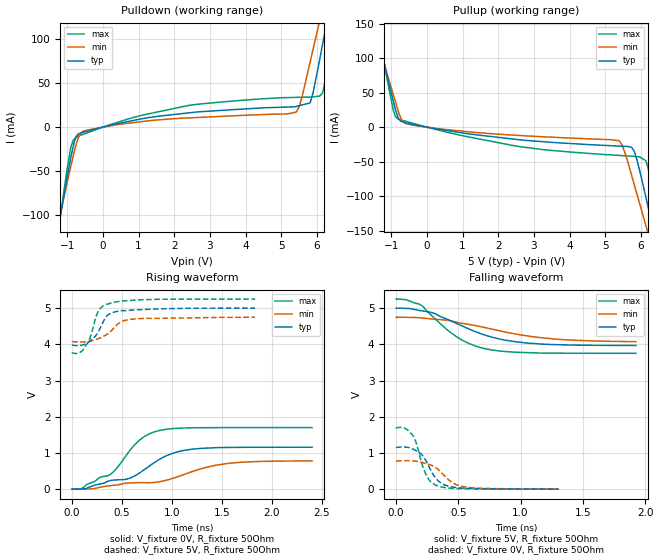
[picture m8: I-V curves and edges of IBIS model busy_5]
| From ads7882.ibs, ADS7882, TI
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|   busy_5 Model
[Model]   busy_5
Model_type   Output
Polarity   Non-Inverting
Vmeas = 2.5
Vref = 2.5
Cref = 20pF
Rref = 50
|   typ   min   max
|   (nom PVT)   (Fast PVT)   (slow PVT)
|C_comp from frequency sweep method (F=1.5MHz)
C_comp   1.072e-12   9.914e-13   1.154e-12
|ON state : BUFFER OUTPUT TURNED HIGH
|C_comp   1.072e-12   9.914e-13   1.154e-12
|OFF state: BUFFER OUTPUT TURNED LOW
|C_comp   1.063e-12   9.642e-13   1.166e-12
|C_comp from LC tank measurement(L=1nH)
|Resonant Frequency(Hz)   6.060e+09   6.040e+09   6.110e+09
|C_comp   6.904e-13   6.950e-13   6.792e-13
|ON state : BUFFER OUTPUT TURNED HIGH
|Resonant Frequency(Hz)   6.060e+09   6.040e+09   6.110e+09
|C_comp   6.904e-13   6.950e-13   6.792e-13
|OFF state: BUFFER IN HIGH IMPEDANCE
|Resonant Frequency   6.010e+09   6.060e+09   5.410e+09
|C_comp   7.020e-13   6.905e-13   8.663e-13
| Where nom  PVT is Nominal Process,  5V,  25C
|   Fast PVT is Strong Process,   5.25V,  -40C
|   Slow PVT is Weak Process,   4.75V,  85C
[Voltage Range]   5   4.75   5.25
|Ambient Temperature   25   85   -40
|Junction Temperature
[Temperature Range]   25   85   -40
[Pullup Reference]   5   4.75   5.25
[Pulldown Reference]   0   0   0
[Power Clamp Reference]   5   4.75   5.25
[GND Clamp Reference]   0   0   0
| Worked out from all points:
|   slope of the pulldown table from 0 to 0.75 V, typ, clamps not added: 112 ohm
|   slope of the pullup table from 0 to 0.75 V, typ, clamps not added: 117 ohm
|   falling waveform, V_fixture 5V, R_fixture 50Ohm: 20-80 % time 455ps typ, 622ps min, 328ps max; typ from 5 V to 3.97 V
|   rising waveform, V_fixture 0V, R_fixture 50Ohm: 20-80 % time 573ps typ, 856ps min, 380ps max; typ from 0 V to 1.16 V
|   rising waveform, V_fixture 5V, R_fixture 50Ohm: 20-80 % time 138ps typ, 182ps min, 112ps max; typ from 3.97 V to 5 V
|   falling waveform, V_fixture 0V, R_fixture 50Ohm: 20-80 % time 125ps typ, 159ps min, 96.5ps max; typ from 1.16 V to 0.001 V
[Pulldown]
|   Voltage   I(typ)   I(min)   I(max)
-5V       -980.4mA   -810.7mA   -1.213A
-1.25V    -113.1mA   -108.5mA   -117.5mA
-905mV    -35.43mA   -45.05mA   -23.42mA
-755mV    -10.91mA   -19.92mA   -12.08mA
-563.5mV  -5.971mA   -4.571mA   -8.317mA
2.361V    15.96mA    10.38mA    24.28mA
5.417V    23.42mA    16.99mA    33.74mA
5.81V     27.46mA    73.68mA    34.14mA
6.072V    75.29mA    119.6mA    35.08mA
6.255V    114.1mA    151.6mA    56.41mA
7.815V    448.6mA    427.9mA    466mA
10V       917.1mA    814.8mA    1.046A
[Pullup]
|   Voltage   I(typ)   I(min)   I(max)
-5V       916mA      771mA      1.109A
-1.25V    103.6mA    101.2mA    104.3mA
-884mV    25.66mA    36.86mA    15.37mA
-800mV    12.74mA    22.42mA    11.62mA
-587.3mV  5.914mA    5.023mA    8.376mA
2.555V    -18.04mA   -11.96mA   -27.82mA
5.388V    -27.44mA   -19.73mA   -40.94mA
5.81V     -34.39mA   -82.4mA    -42.28mA
6.188V    -112.1mA   -151.2mA   -56.41mA
6.265V    -129.5mA   -165.3mA   -74.45mA
7.29V     -363.4mA   -356.3mA   -367.1mA
10V       -986.8mA   -861.2mA   -1.153A
[Ramp]
R_load = 50
|   typ   min   max
dV/dt_r   0.694763/5.72602e-10   0.468296/8.56219e-10   1.01977/3.8037e-10
dV/dt_f   0.61811/4.56691e-10   0.408104/6.31351e-10   0.898003/3.28003e-10
[Falling Waveform]
V_fixture = 5V
V_fixture_min = 4.75V
V_fixture_max = 5.25V
R_fixture = 50Ohm
|   Time   V(typ)   V(min)   V(max)
0s        5V         4.75V      5.25V
78.25ps   4.996V     4.75V      5.236V
202.6ps   4.93V      4.732V     5.081V
302.8ps   4.862V     4.699V     4.74V
483.5ps   4.584V     4.613V     4.216V
579.5ps   4.435V     4.556V     4.033V
723.5ps   4.248V     4.458V     3.876V
873.4ps   4.12V      4.345V     3.805V
1.161ns   4.011V     4.189V     3.762V
1.927ns   3.972V     4.076V     3.754V
[Rising Waveform]
V_fixture = 0V
V_fixture_min = 0V
V_fixture_max = 0V
R_fixture = 50Ohm
|   Time   V(typ)   V(min)   V(max)
0s        2.197nV    6.551nV    2.052nV
90.57ps   3.134mV    -1.357uV   11.49mV
280ps     141.1mV    50.58mV    325.7mV
377.5ps   232.9mV    92.98mV    397mV
553.8ps   281.4mV    166.8mV    977.6mV
675.5ps   447.5mV    178.7mV    1.357V
867.5ps   812.5mV    201.2mV    1.616V
1.113ns   1.066V     398.5mV    1.687V
1.543ns   1.15V      703.2mV    1.699V
2.4ns     1.158V     780.5mV    1.7V
[Rising Waveform]
V_fixture = 5V
V_fixture_min = 4.75V
V_fixture_max = 5.25V
R_fixture = 50Ohm
|   Time   V(typ)   V(min)   V(max)
0s        3.969V     4.068V     3.753V
67.5ps    3.965V     4.066V     3.762V
122.4ps   3.997V     4.068V     3.9V
177.8ps   4.087V     4.085V     4.172V
263.1ps   4.353V     4.158V     4.923V
336.2ps   4.744V     4.253V     5.099V
386.9ps   4.858V     4.361V     5.138V
482.4ps   4.924V     4.611V     5.189V
607.7ps   4.946V     4.696V     5.218V
1.831ns   4.999V     4.748V     5.25V
[Falling Waveform]
V_fixture = 0V
V_fixture_min = 0V
V_fixture_max = 0V
R_fixture = 50Ohm
|   Time   V(typ)   V(min)   V(max)
0s        1.158V     782.7mV    1.7V
67.5ps    1.165V     788.5mV    1.688V
132.9ps   1.111V     783.1mV    1.488V
160.1ps   1.059V     772.1mV    1.291V
206.2ps   951.6mV    741mV      716.9mV
246.7ps   737.4mV    700.7mV    354.2mV
336.2ps   236.4mV    547.4mV    86.01mV
431.2ps   74.66mV    229.9mV    30.05mV
542.2ps   29.99mV    69.99mV    12.5mV
1.305ns   1.028mV    4.08mV     435.5uV
